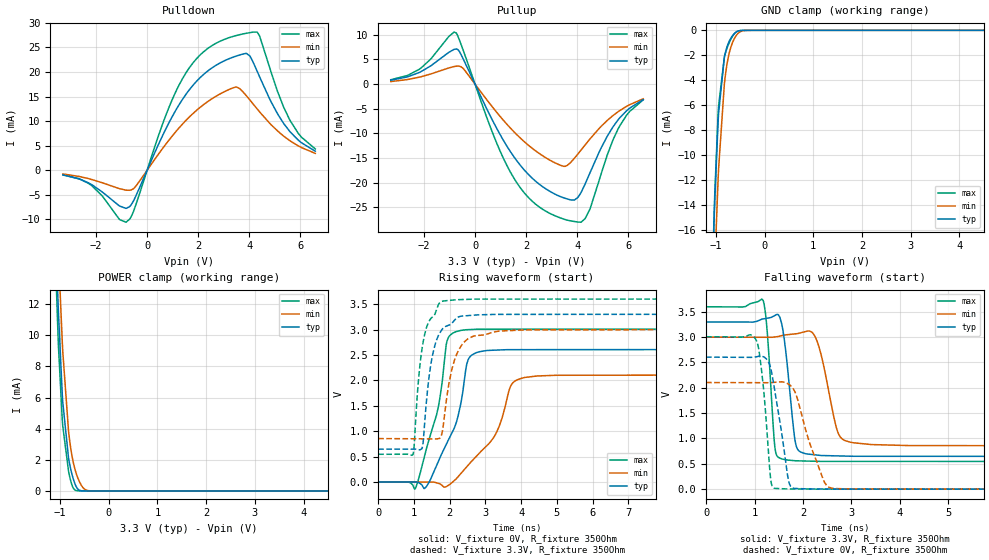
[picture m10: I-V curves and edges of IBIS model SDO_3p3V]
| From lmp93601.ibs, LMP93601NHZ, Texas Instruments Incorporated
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|   Model SDO_3p3V
[Model]   SDO_3p3V
Model_type   3-state
Polarity   Non-Inverting
Vmeas = 1.65
Vref = 3.3
Cref = 15pF
Rref = 350
|   typ   min   max
|   (nom PVT)   (fast PVT)   (slow PVT)
C_comp   0.1267p   0.1173p   0.1344p
|C_comp (ON state)   0.1308p   0.1205p   0.1360p
|C_comp (OFF state)   0.1267p   0.1173p   0.1344p
[Voltage Range]   3.3   3   3.6
[Temperature Range]   27   125   -25
[Pullup Reference]   3.3   3   3.6
[Pulldown Reference]   0   0   0
[Power Clamp Reference]   3.3   3   3.6
[GND Clamp Reference]   0   0   0
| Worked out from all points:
|   slope of the pulldown table from 0 to 0.495 V, typ, clamps not added: 85.3 ohm
|   slope of the pullup table from 0 to 0.495 V, typ, clamps not added: 91.8 ohm
|   GND clamp passes 1 mA (typ) near -0.74 V on its own axis
|   POWER clamp passes 1 mA (typ) near -0.75 V on its own axis
|   falling waveform, V_fixture 3.3V, R_fixture 350Ohm: 20-80 % time 168ps typ, 276ps min, 121ps max; typ from 3.3 V to 0.647 V
|   rising waveform, V_fixture 0V, R_fixture 350Ohm: 20-80 % time 671ps typ, 989ps min, 527ps max; typ from 0 V to 2.61 V
|   rising waveform, V_fixture 3.3V, R_fixture 350Ohm: 20-80 % time 320ps typ, 383ps min, 289ps max; typ from 0.647 V to 3.3 V
|   falling waveform, V_fixture 0V, R_fixture 350Ohm: 20-80 % time 252ps typ, 417ps min, 161ps max; typ from 2.61 V to 0 V
[Pulldown]
|   Voltage   I(typ)   I(min)   I(max)
-3.3V     -961.3uA   -755.9uA   -885uA
-2.171V   -2.935mA   -1.882mA   -3.131mA
-825mV    -7.763mA   -4.054mA   -10.57mA
-528mV    -6.183mA   -3.73mA    -8.294mA
858mV     9.683mA    6.143mA    12.82mA
1.601V    16mA       10.55mA    20.43mA
2.412V    20.34mA    14.1mA     24.9mA
3.472V    23.19mA    16.93mA    27.37mA
4.165V    21.85mA    13.41mA    28.11mA
4.402V    19.06mA    11.91mA    27.37mA
5.59V     7.894mA    6.019mA    10.23mA
6.59V     3.865mA    3.424mA    4.332mA
[GND Clamp]
|   Voltage   I(typ)   I(min)   I(max)
-3.3V     -527.6mA   -476.3mA   -564.6mA
-1.043V   -16.11mA   -21.29mA   -15.77mA
-1.033V   -14.89mA   -20.1mA    -14.46mA
-1.023V   -13.73mA   -18.94mA   -13.22mA
-953.7mV  -7.328mA   -11.95mA   -6.701mA
-943.8mV  -6.661mA   -11.12mA   -6.066mA
-825mV    -2.156mA   -4.294mA   -2.143mA
-775.5mV  -1.386mA   -2.819mA   -1.488mA
-716.1mV  -800.6uA   -1.682mA   -910.5uA
-547.8mV  -68.6uA    -257.2uA   -62.33uA
-270.6mV  -24.98nA   -610.3nA   -2.234nA
6.59V     0A         0A         0A
[Pullup]
|   Voltage   I(typ)   I(min)   I(max)
-3.3V     779.5uA    513.2uA    885.8uA
-2.142V   2.469mA    1.457mA    3.169mA
-735.9mV  7.127mA    3.632mA    10.38mA
-468.6mV  5.154mA    3.192mA    6.929mA
838.2mV   -8.874mA   -5.653mA   -11.84mA
1.64V     -15.58mA   -10.27mA   -20.04mA
2.501V    -20.24mA   -14.02mA   -24.87mA
3.462V    -23.05mA   -16.67mA   -27.36mA
4.036V    -22.95mA   -14.15mA   -27.99mA
4.501V    -18.03mA   -11.15mA   -25.38mA
5.61V     -7.225mA   -5.591mA   -9.06mA
6.59V     -3.139mA   -2.986mA   -3.199mA
[POWER Clamp]
|   Voltage   I(typ)   I(min)   I(max)
-3.3V     344.8mA    311.7mA    366.2mA
-1.073V   15.06mA    18.74mA    12.92mA
-1.063V   14.12mA    17.85mA    11.96mA
-1.043V   12.34mA    16.14mA    10.17mA
-1.033V   11.5mA     15.31mA    9.349mA
-943.8mV  5.705mA    8.97mA     4.174mA
-825mV    2.109mA    3.84mA     1.264mA
-755.7mV  1.084mA    2.278mA    386.9uA
-676.5mV  333.9uA    1.216mA    33.27uA
-547.8mV  7.035uA    293.2uA    408.9nA
-409.2mV  51.4nA     13.95uA    0A
6.59V     0A         0A         0A
[Ramp]
R_load = 350
|   typ   min   max
dV/dt_r   1.56369/6.71743e-10   1.26282/9.87959e-10   1.80514/5.2806e-10
dV/dt_f   1.59202/1.68153e-10   1.28666/2.7569e-10   1.83225/1.20765e-10
[Falling Waveform]
V_fixture = 3.3V
V_fixture_min = 3V
V_fixture_max = 3.6V
R_fixture = 350Ohm
C_fixture = 0F
|   Time   V(typ)   V(min)   V(max)
0s        3.3V       3V         3.6V
1.178ns   3.36V      2.998V     3.722V
1.417ns   3.426V     3.004V     853.4mV
1.555ns   3.284V     3.029V     599.8mV
1.832ns   983.2mV    3.064V     561.7mV
2.034ns   704.8mV    3.106V     555.7mV
2.291ns   672.7mV    2.92V      549.6mV
2.715ns   656.6mV    1.137V     548.1mV
2.964ns   650.8mV    930.2mV    548mV
10ns      646.6mV    855.6mV    546.2mV
[Rising Waveform]
V_fixture = 0V
V_fixture_min = 0V
V_fixture_max = 0V
R_fixture = 350Ohm
C_fixture = 0F
|   Time   V(typ)   V(min)   V(max)
0s        5.853nV    12.82nV    8.767nV
1.046ns   523.4uV    -203.4uV   -118.7mV
1.355ns   -82.58mV   -263.6uV   670.7mV
1.683ns   403.9mV    -25.29mV   1.477V
1.924ns   768.5mV    -82.41mV   2.768V
2.112ns   1.036V     18.95mV    2.939V
2.546ns   2.444V     354.9mV    2.999V
3.258ns   2.595V     905.5mV    3.007V
3.885ns   2.605V     2.01V      3.007V
10ns      2.606V     2.105V     3.009V
[Rising Waveform]
V_fixture = 3.3V
V_fixture_min = 3V
V_fixture_max = 3.6V
R_fixture = 350Ohm
C_fixture = 0F
|   Time   V(typ)   V(min)   V(max)
0s        646.6mV    855.6mV    546.2mV
982.6ps   647.3mV    851.5mV    558.2mV
1.13ns    637.9mV    850.9mV    2.026V
1.263ns   829.2mV    850.4mV    2.777V
1.466ns   2.279V     849.6mV    3.21V
1.768ns   2.981V     913mV      3.55V
1.977ns   3.087V     1.922V     3.573V
2.139ns   3.187V     2.407V     3.584V
2.659ns   3.283V     2.868V     3.598V
10ns      3.3V       3V         3.6V
[Falling Waveform]
|Gnd
V_fixture = 0V
V_fixture_min = 0V
V_fixture_max = 0V
R_fixture = 350Ohm
C_fixture = 0F
|   Time   V(typ)   V(min)   V(max)
0s        2.606V     2.105V     3.009V
1.046ns   2.614V     2.102V     2.918V
1.185ns   2.612V     2.101V     1.991V
1.331ns   2.395V     2.103V     211.7mV
1.401ns   2.04V      2.108V     19.85mV
1.697ns   191.1mV    2.076V     5.426mV
1.807ns   16.66mV    1.969V     4.554mV
2.416ns   3.417mV    195.7mV    570.5uV
2.589ns   2.334mV    20.2mV     557.5uV
10ns      -14.37nV   30.87nV    81.91nV
